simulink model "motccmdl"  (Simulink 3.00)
settings: Solver=ode45  StartTime=0.0  StopTime=10.0  RelTol=1e-3
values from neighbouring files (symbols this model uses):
  b = 0.001    [motcc.m]
  J = 0.03    [motcc.m]
  ke = 0.5    [motcc.m]
  L = 0.001    [motcc.m]
  R = 1    [motcc.m]
  t0 = 1    [motcc.m]
  V0 = 100    [motcc.m]
undefined symbols (not defined in the file or in its folder): Ce
libraries: cstblocks x2

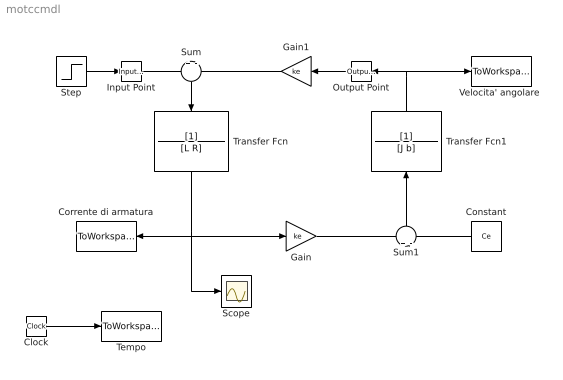
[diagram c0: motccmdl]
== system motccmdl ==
  Clock : Clock
  Constant : Constant  Orientation=left  Value=Ce
  Corrente di armatura : ToWorkspace  VariableName=Ia  SampleTime=-1  SaveFormat=Matrix
  Gain : Gain  Gain=ke  SaturateOnIntegerOverflow=on
  Gain1 : Gain  Orientation=left  Gain=ke  SaturateOnIntegerOverflow=on
  Input Point : cstblocks/Input Point  PerturbationValue=0
  Output Point : cstblocks/Output Point  Orientation=left  SigprobeOutputIndex=1
  Scope : Scope
  Step : Step  Time=t0  Before=0  After=V0  SampleTime=0
  Sum : Sum  Orientation=down  Inputs=+|-  SaturateOnIntegerOverflow=on
  Sum1 : Sum  Orientation=up  Inputs=+|-  SaturateOnIntegerOverflow=on
  Tempo : ToWorkspace  VariableName=t  SampleTime=-1  SaveFormat=Matrix
  Transfer Fcn : TransferFcn  Orientation=down  Numerator=[1]  Denominator=[L R]
  Transfer Fcn1 : TransferFcn  Orientation=up  Numerator=[1]  Denominator=[J b]
  "Velocita' angolare " : ToWorkspace  VariableName=wm  SampleTime=-1  SaveFormat=Matrix
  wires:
  Sum/1 -> Transfer Fcn/1
  Constant/1 -> Sum1/2
  Sum1/1 -> Transfer Fcn1/1
  Gain/1 -> Sum1/1
  Gain1/1 -> Sum/2
  Transfer Fcn/1 -> Corrente di armatura/1, Gain/1, Scope/1
  Transfer Fcn1/1 -> "Velocita' angolare "/1, Output Point/1
  Clock/1 -> Tempo/1
  Step/1 -> Input Point/1
  Input Point/1 -> Sum/1
  Output Point/1 -> Gain1/1
